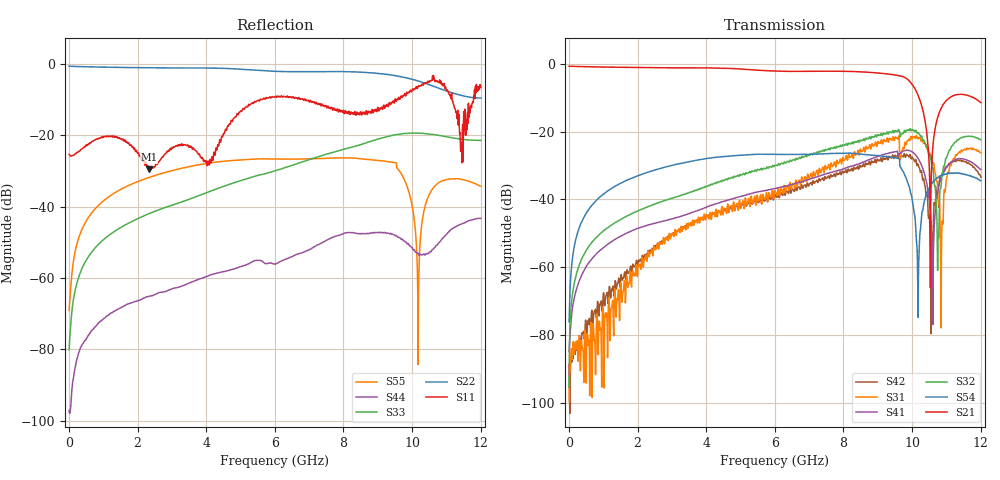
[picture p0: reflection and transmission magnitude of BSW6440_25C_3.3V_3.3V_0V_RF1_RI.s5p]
!	Test time	=	2022-08-08 18:02
!	Product	=	BSW6440
!	Temp	=	25C
!	VDD	=	3.3
!	Control_High	=	3.3
!	Control_Low	=	0
!	Logic	=	RF1
!	Porrt1	=	RFC
!	Porrt2	=	RF1
!	Porrt3	=	RF2
!	Porrt4	=	RF3
!	Porrt5	=	RF4
!	V1(LS)	=	0
!	V2(CTRL)	=	X
!	V3	=	X
!	V4	=	X
#	Hz	S	RI	R	50
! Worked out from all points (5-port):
!   1201 points, 5 MHz to 12.01 GHz, reference 50 ohm
!   strongest paths, dB at 5 MHz, 3.005 GHz, 6.005 GHz, 9.005 GHz, 12.01 GHz:
!     S21: -0.6, -1.1, -2.1, -2.7, -11.4
!     S54: -76.1, -29.9, -26.7, -27.0, -34.5
!     S32: -95.3, -39.6, -29.9, -20.9, -22.4
!     S41: -84.8, -45.7, -36.7, -27.3, -31.2
!     S31: -88.9, -50.5, -37.4, -22.8, -26.2
!     S42: -88.6, -50.3, -38.7, -28.4, -33.4
!   lowest |S11| = -29.6 dB at 2.335 GHz (marker M1), VSWR 1.07, Z = 48.3 + j2.8 ohm
!   |S11| at or under -10 dB: start of sweep to 5.569 GHz; 6.884 GHz to 9.501 GHz (2.617 GHz wide, 31.9 % of centre); 11.17 GHz to 11.79 GHz (621.3 MHz wide, 5.41 % of centre)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
